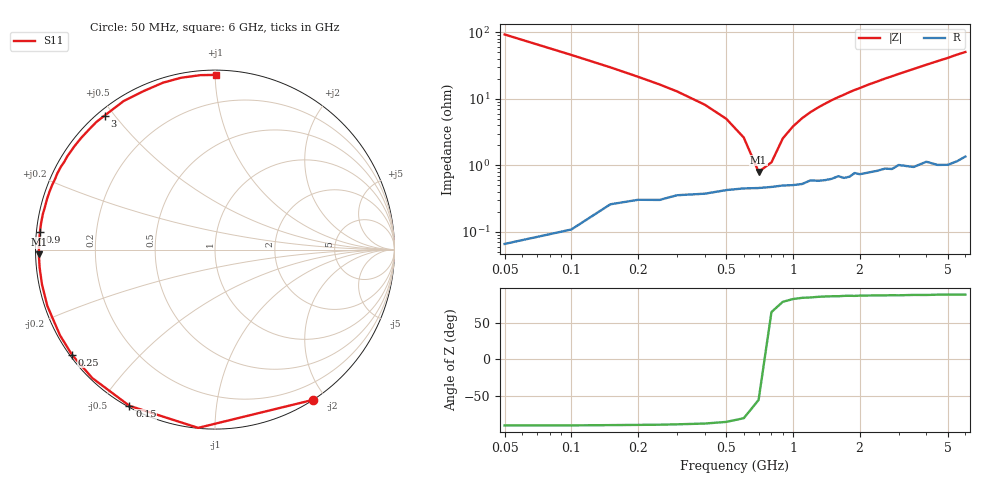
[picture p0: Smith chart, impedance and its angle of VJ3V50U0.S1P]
! Infineon Technologies  Discrete & RF Semiconductors
! BB 914
! Si Tuning Diode in SOT23
! VR = 3.5 V
! S-Parameters:  July  1999
# GHz  S  MA  R  50
!  f  S11
! GHz  MAG  ANG
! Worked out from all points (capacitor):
!   34 points, 50 MHz to 6 GHz, reference 50 ohm
!   read as one part to ground: C = 34.3 pF near 50 MHz
!   lowest |Z| = 798 mohm at 700 MHz (marker M1)
!   series resonance near 739.5 MHz, so ESL is about 1.3 nH
!   S11 on the Smith chart (normalised r, x): 50 MHz: 0.00, -1.85; 150 MHz: 0.01, -0.59; 250 MHz: 0.01, -0.33; 900 MHz: 0.01, +0.05; 3 GHz: 0.02, +0.47; 6 GHz: 0.03, +1.01
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0.05  0.9994 -56.9
0.1  0.9976 -95.4
0.15  0.9923 -118.7
0.2  0.9898 -133.7
0.25  0.9891 -143.7
0.3  0.9867 -151.1
0.4  0.9855 -161.5
0.5  0.9833 -168.6
0.6  0.9822 -174.1
0.7  0.9819 -178.5
0.8  0.9812 177.7
0.9  0.9803 174.3
1.2  0.9769 165.7
1.5  0.976 158.4
1.6  0.974 156.2
1.7  0.9757 154.1
1.9  0.9718 149.7
2.2  0.9721 143.7
2.4  0.9711 140.1
2.6  0.9697 136.3
2.8  0.9708 133.0
3  0.9674 129.5
3.5  0.9716 121.6
4  0.9686 114.1
4.5  0.974 107.3
5  0.9759 101.2
5.5  0.9753 94.8
6  0.9734 89.6
